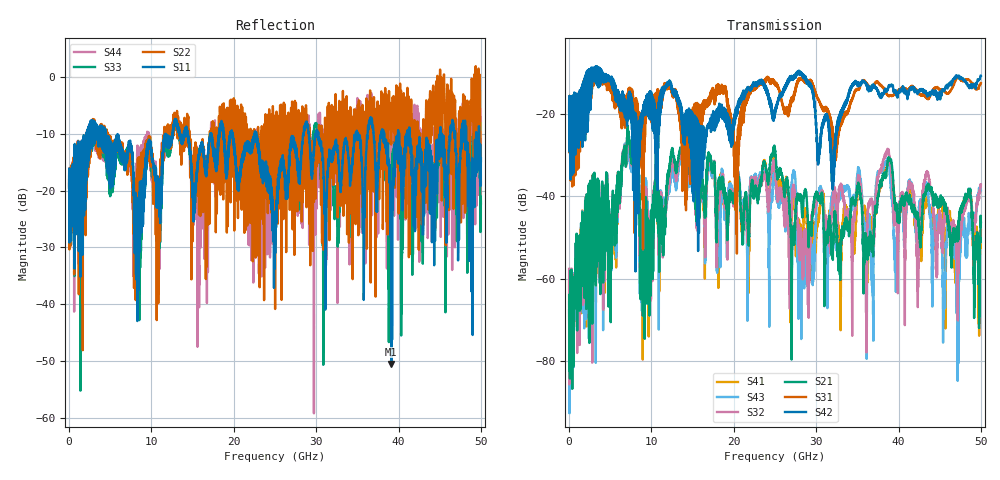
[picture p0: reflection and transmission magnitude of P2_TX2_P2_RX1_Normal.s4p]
!Keysight Technologies,N5225B,MY57041031,A.13.20.10
!Date: Friday, May 31, 2019 11:27:24
!Correction: S11(Full 4 Port(1,2,3,4))
!S12(Full 4 Port(1,2,3,4))
!S13(Full 4 Port(1,2,3,4))
!S14(Full 4 Port(1,2,3,4))
!S21(Full 4 Port(1,2,3,4))
!S22(Full 4 Port(1,2,3,4))
!S23(Full 4 Port(1,2,3,4))
!S24(Full 4 Port(1,2,3,4))
!S31(Full 4 Port(1,2,3,4))
!S32(Full 4 Port(1,2,3,4))
!S33(Full 4 Port(1,2,3,4))
!S34(Full 4 Port(1,2,3,4))
!S41(Full 4 Port(1,2,3,4))
!S42(Full 4 Port(1,2,3,4))
!S43(Full 4 Port(1,2,3,4))
!S44(Full 4 Port(1,2,3,4))
!S4P File: Measurements: <S11,S12,S13,S14>,
!<S21,S22,S23,S24>,
!<S31,S32,S33,S34>,
!<S41,S42,S43,S44>:
# Hz S  dB  R 50.0
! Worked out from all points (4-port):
!   5000 points, 10 MHz to 50 GHz, reference 50 ohm
!   strongest paths, dB at 10 MHz, 12.51 GHz, 25.01 GHz, 37.51 GHz, 50 GHz:
!     S42: -19.5, -14.3, -20.1, -14.6, -10.7
!     S31: -19.4, -14.9, -13.0, -12.4, -12.6
!     S21: -67.7, -28.9, -29.2, -39.6, -46.4
!     S32: -57.6, -31.3, -33.6, -35.3, -37.2
!     S43: -65.7, -34.0, -36.4, -34.0, -38.5
!     S41: -60.5, -31.4, -32.2, -39.5, -48.1
!   lowest |S11| = -50.5 dB at 39.13 GHz (marker M1), VSWR 1.01, Z = 50.2 + j0.17 ohm
!   |S11| at or under -10 dB: 4.481 GHz to 11.72 GHz (7.238 GHz wide, 89.4 % of centre); 22.73 GHz to 28.43 GHz (5.703 GHz wide, 22.3 % of centre); 30.26 GHz to 34.82 GHz (4.557 GHz wide, 14 % of centre)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
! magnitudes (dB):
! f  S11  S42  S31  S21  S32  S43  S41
! 10 MHz  -19.1  -19.5  -19.4  -67.7  -57.6  -65.7  -60.5
! 7.23 GHz  -12.0  -17.7  -16.8  -24.3  -25.6  -26.6  -25.4
! 8.84 GHz  -21.4  -22.3  -26.4  -45.3  -53.4  -56.7  -53.7
! 13.79 GHz  -10.8  -22.9  -22.9  -27.4  -28.9  -30.0  -28.7
! 29.08 GHz  -9.8  -13.1  -12.3  -52.3  -58.5  -54.5  -54.6
! 39.13 GHz  -50.5  -13.0  -15.6  -31.8  -34.4  -39.6  -33.1
! 50 GHz  -14.3  -10.7  -12.6  -46.4  -37.2  -38.5  -48.1
